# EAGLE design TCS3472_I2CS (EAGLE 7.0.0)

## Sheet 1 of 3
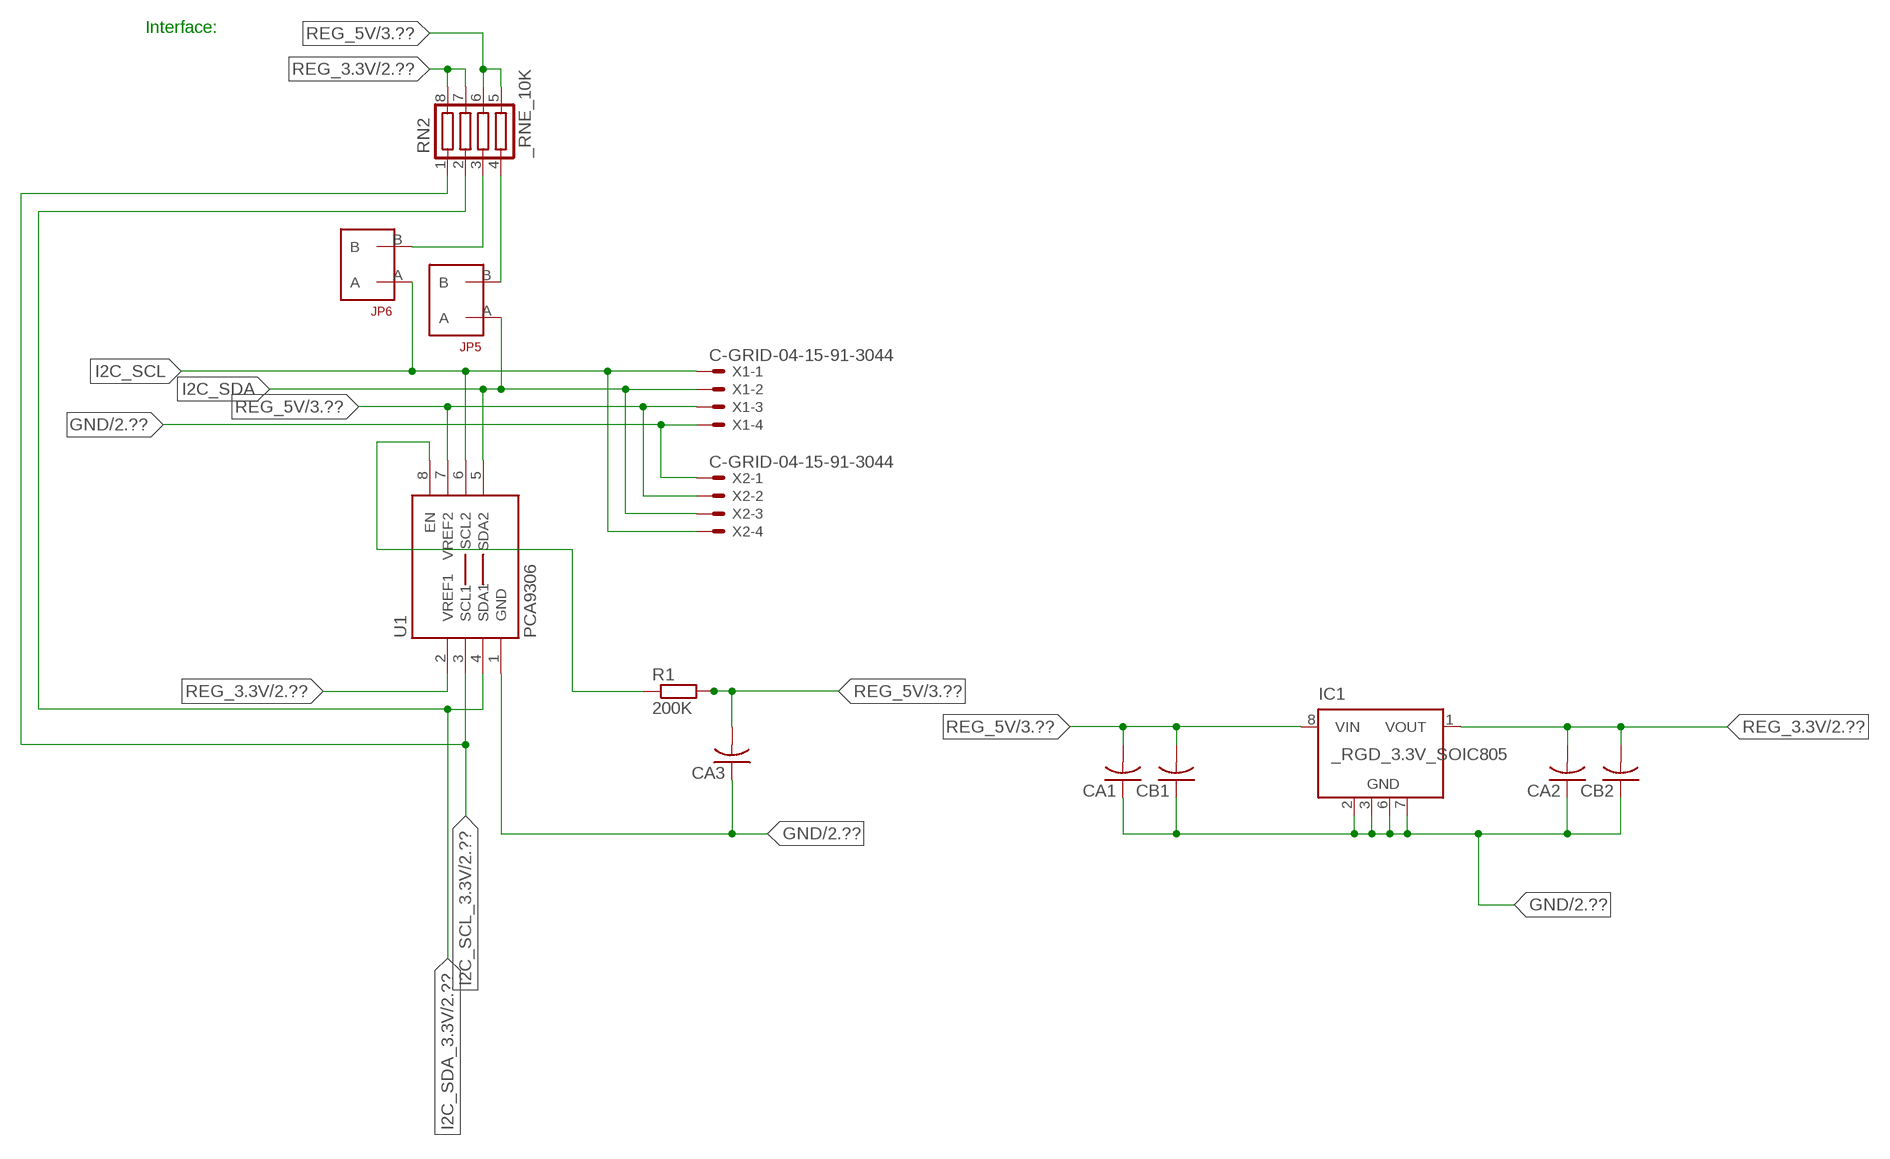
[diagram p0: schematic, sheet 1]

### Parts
CA1  CC1206KRX7R9BB104  [.1UF]
CA2  CC1206KRX7R9BB104  [.1UF]
CA3  CC1206KRX7R9BB104  [.1UF]
CB1  TMK316F106ZL-TC1206K  [TMK316F106ZL-T]
CB2  TMK316F106ZL-TC1206K  [TMK316F106ZL-T]
IC1  _RGD_3.3V_SOIC805  [_RGC_3.3V_SOIC8]
JP5  JUMPER_1X2_2MM  [JUMPER_1X2_2MM]
JP6  JUMPER_1X2_2MM  [JUMPER_1X2_2MM]
R1  200K  RESISTOR_SMT-0603  [R603]
RN2  _RNE_10K  [RNE]
U1  PCA9306  PCA9306_NCD  [PSOP-8]
X1  C-GRID-04-15-91-3044  [15-91-04]
X2  C-GRID-04-15-91-3044  [15-91-04]

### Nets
GND: CA1.1 CA2.1 CA3.1 CB1.1 CB2.1 IC1.2(GND) IC1.3(GND) IC1.6(GND) IC1.7(GND) U1.1(GND) X1.4 X2.1 ; also sheet 2,3
I2C_SCL: JP6.A U1.6(SCL2) X1.1 X2.4
I2C_SCL_3.3V: RN2.1 U1.3(SCL1) ; also sheet 2
I2C_SDA: JP5.A U1.5(SDA2) X1.2 X2.3
I2C_SDA_3.3V: RN2.2 U1.4(SDA1) ; also sheet 2
N$1: JP6.B RN2.3
N$2: JP5.B RN2.4
N$23: R1.1 U1.8(EN)
REG_3.3V: CA2.2 CB2.2 IC1.1(VOUT) RN2.7 RN2.8 U1.2(VREF1) ; also sheet 2
REG_5V: CA1.2 CA3.2 CB1.2 IC1.8(VIN) R1.2 RN2.5 RN2.6 U1.7(VREF2) X1.3 X2.2 ; also sheet 3
Unconnected: IC1.4(NC) IC1.5(NC)

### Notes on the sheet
- Interface:

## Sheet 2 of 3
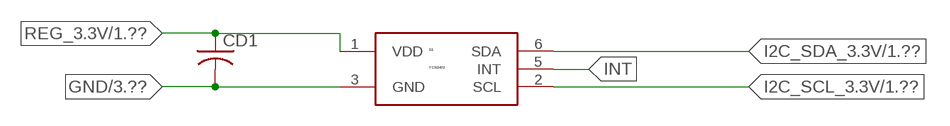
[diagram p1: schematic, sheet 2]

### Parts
CD1  CC1206KRX7R9BB103C1206K  [CC1206KRX7R9BB103]
S1  TCS3472  [FN-6]

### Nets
GND: CD1.2 S1.3(GND) ; also sheet 1,3
I2C_SCL_3.3V: S1.2(SCL) ; also sheet 1
I2C_SDA_3.3V: S1.6(SDA) ; also sheet 1
INT: S1.5(INT)
REG_3.3V: CD1.1 S1.1(VDD) ; also sheet 1

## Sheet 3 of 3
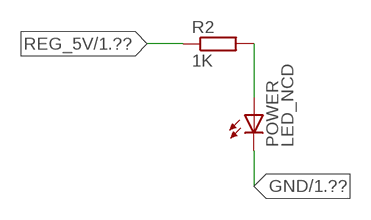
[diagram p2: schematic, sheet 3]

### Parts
POWER  LED_NCD  [CHIPLED_0603]
R2  1K  RESISTOR_SMT-0402  [R402]

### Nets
GND: POWER.C ; also sheet 1,2
N$4: POWER.A R2.2
REG_5V: R2.1 ; also sheet 1

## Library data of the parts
CA1-CA3 = NCD_ULTIMATE_LIBRARY:CC1206KRX7R9BB104: Capacitor CA .1uF 50V SMT C1206K CC1206KRX7R9BB104
CB1 CB2 = NCD_ULTIMATE_LIBRARY:TMK316F106ZL-T: Capacitor CB 10uF SMT 1206 TMK316F106ZL-T
CD1 = NCD_ULTIMATE_LIBRARY:CC1206KRX7R9BB103: Capacitor CD .01uF SMT CC1206KRX7R9BB103 1206
IC1 = NCD_ULTIMATE_LIBRARY:_RGD_3.3V_SOIC8: Regulator Linear 3.3V Chip Positive VOLTAGE REGULATOR Digikey 497-1199-2-ND/L78L33ACD13TR
JP5 JP6 = NCD_ULTIMATE_CONNECTORS:JUMPER_1X2_2MM
POWER = NCD_ULTIMATE_LIBRARY:LED_NCD: LED Digikey 754-1132-2-ND/APT2012SRCPRV
R1 R2 = NCD_ULTIMATE_LIBRARY:RESISTOR_SMT: NCD Resistor
RN2 = NCD_ULTIMATE_LIBRARY:_RNE_10K: Resistor Array RNE SMT 10K x 4 Single Resistor Source: http://www.ctscorp.com/components/Datasheets/CTSChipArrayDs.pdf Digikey 742C083103JPTR-ND/742C083103JP; OC_FARNELL: unknown; OC_NEWARK: unknown
S1 = NCD_ULTIMATE_bhaskar:TCS3472: Color Sensor Digikey TCS34725FNTR-ND/TCS34725FN
U1 = NCD_ULTIMATE_LIBRARY:PCA9306_NCD: NCD Bidirectional I2C level shifter. NOT compatible with all available part number pinout schemes- DOUBLE CHECK!!!; PROD_ID: IC-10023
X1 X2 = NCD_ULTIMATE_CONNECTORS:C-GRID-04: CONNECTOR 4-Pos I2C wire to board 2.54 mm (0.100") pitch header Digikey WM1342-ND/0015912045; OC_FARNELL: unknown; OC_NEWARK: unknown

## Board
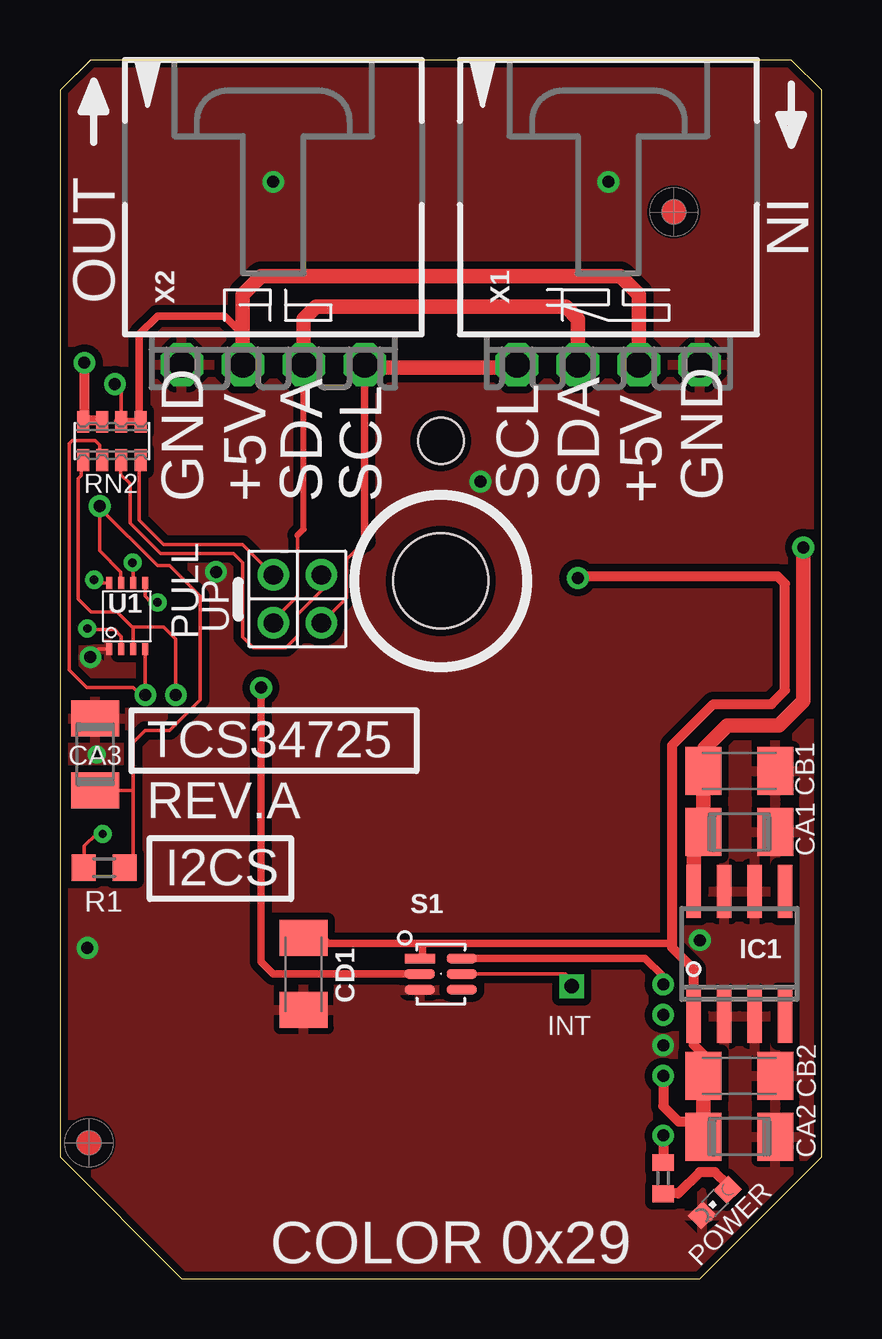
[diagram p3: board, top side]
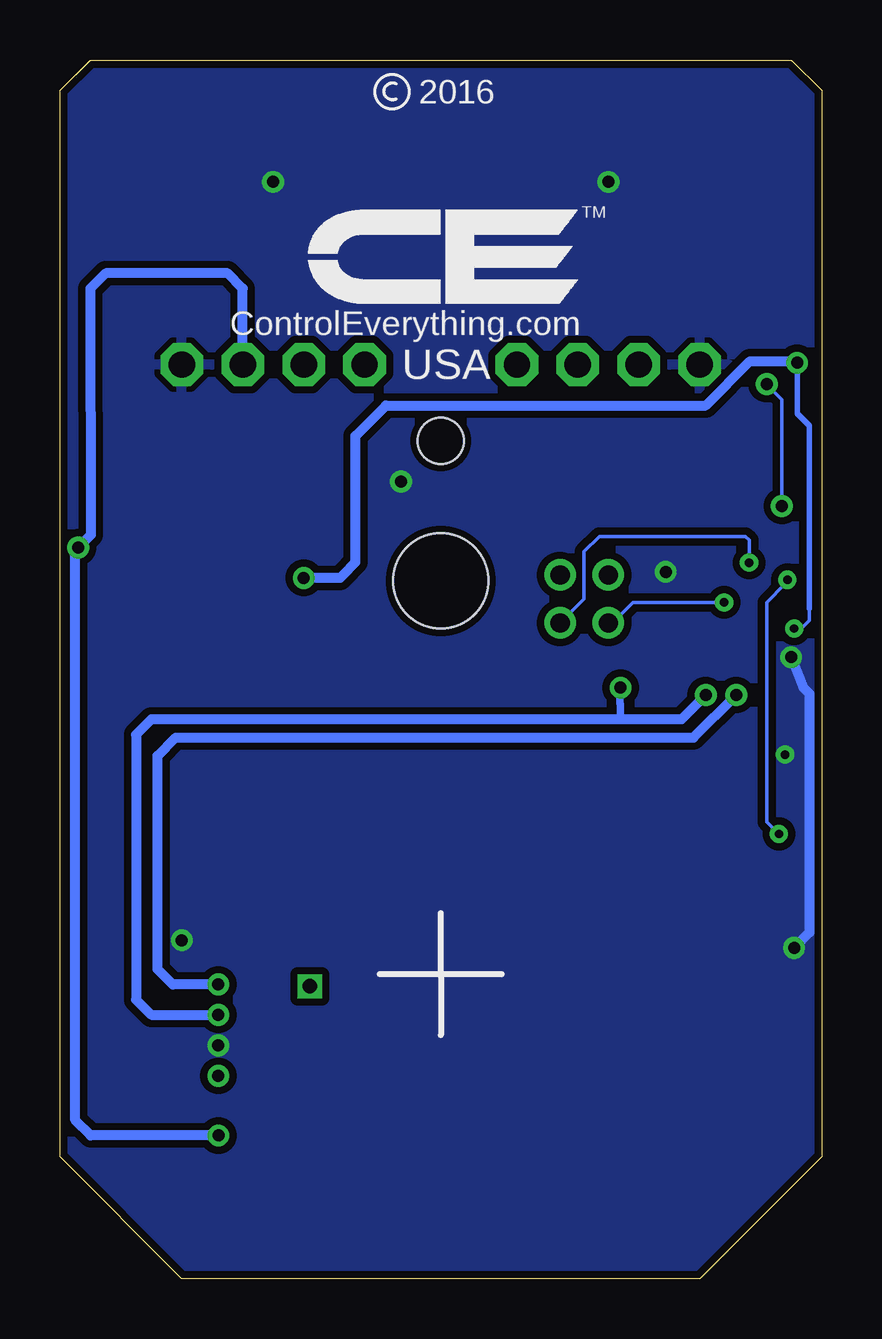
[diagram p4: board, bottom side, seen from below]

Size 31.75 x 50.8 mm. Coordinates in mm from the lower left corner, seen from the top.
Outline: 32 segments
Copper layers (1*16): Top 0.035mm / dielectric 1.5mm / Bottom 0.035mm
Design rules "default": minimum track width 5mil, minimum drill 24mil, track to track 5mil, track to pad 5mil, pad to pad 5mil, via to via 5mil, smd to smd 5mil, copper to edge 10mil, drill to drill 8mil, minimum pad ring 10mil, minimum via ring 8mil, stop-mask expansion 2mil, vias tented up to drill 0mil, thermal gap 10mil
Holes 3.96 mm at 15.88,29.08
Holes 1.91 mm at 15.88,34.93

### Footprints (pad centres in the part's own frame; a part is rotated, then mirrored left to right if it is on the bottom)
.1UF = smd 1.5 x 2: 1 -1.5,0; 2 1.5,0
TMK316F106ZL-T = smd 1.5 x 2: 1 -1.5,0; 2 1.5,0
CC1206KRX7R9BB103 = smd 1.5 x 2: 1 -1.5,0; 2 1.5,0
_RGC_3.3V_SOIC8 = smd 0.6 x 2.2: 1 -1.905,-2.6; 2 -0.635,-2.6; 3 0.635,-2.6; 4 1.905,-2.6; 5 1.905,2.6; 6 0.635,2.6; 7 -0.635,2.6; 8 -1.905,2.6
JUMPER_1X2_2MM = drill 0.8: A 0,2; B 0,0
CHIPLED_0603 = smd 0.8 x 0.876: A 0,-0.75; C 0,0.75
R603 = smd 1 x 1.1: 1 -0.85,0; 2 0.85,0
R402 = smd 0.7 x 0.9: 1 -0.65,0; 2 0.65,0
RNE = smd 0.5 x 0.9: 1 -1.2,-0.8; 2 -0.4,-0.8; 3 0.4,-0.8; 4 1.2,-0.8; 5 1.2,0.8; 6 0.4,0.8; 7 -0.4,0.8; 8 -1.2,0.8
FN-6 = smd 1.25 x 0.4: 1 -0.875,0.65; 2 -0.875,0; 3 -0.875,-0.65; 4 0.875,-0.65; 5 0.875,0; 6 0.875,0.65
PSOP-8 = smd 0.25 x 0.5: 1 -0.73,-1.37; 2 -0.23,-1.37; 3 0.27,-1.37; 4 0.77,-1.37; 5 0.77,1.38; 6 0.27,1.38; 7 -0.23,1.38; 8 -0.73,1.38
15-91-04 = drill 1.1 pad 1.778 octagon: 1 -3.81,-7.62; 2 -1.27,-7.62; 3 1.27,-7.62; 4 3.81,-7.62

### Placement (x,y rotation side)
CA1  28.32,18.62 180 top
CA2  28.32,5.92 180 top
CA3  1.46,21.86 270 top
CB1  28.32,21.16 180 top
CB2  28.32,8.46 180 top
CD1  10.16,12.7 270 top
IC1  28.32,13.54 0 top
JP5  8.89,29.34 180 top
JP6  10.9,29.34 180 top
POWER  27.3,3.18 135 top
R1  1.84,17.13 0 top
R2  25.15,4.19 270 top
RN2  2.16,34.93 0 top
S1  15.88,12.7 0 top
U1  2.79,27.61 0 top
U$5  [VISION_REF10]  1.21,5.66 90 top
U$28  [VISION_REF10]  25.59,44.46 90 top
X1  22.86,45.72 0 top
X2  8.89,45.72 0 top

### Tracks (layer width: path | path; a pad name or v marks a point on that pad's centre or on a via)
GND  (via drill 0.35, 0.5)
  Top 0.152: CA3.1 1.52,23.42 1.52,23.62 | v1.27,25.91 1.6,26.24 U1.1
  Bottom 0.406: v1.27,25.91 0.76,24.64 0.51,24.38 0.51,14.43 v1.15,13.79
  other vias: 8.89,45.72 22.86,45.72 25.15,9.73 17.53,33.22 26.67,14.11 6.5,29.46 1.52,21.84
  pour Bottom (isolate 0.305): -0.64,5.08 -0.64,49.53 1.27,51.44 30.48,51.44 32.38,49.53 32.38,5.08 26.67,-0.63 5.08,-0.63
  pour Top (isolate 0.305): 4.45,-1.27 -1.27,4.45 -1.27,50.17 0.64,52.07 31.11,52.07 33.02,50.17 33.02,4.45 27.3,-1.27
I2C_SCL  (via drill 0.35)
  Top 0.152: 12.7,30.73 11.94,29.97 11.94,28.38 JP6.A | v3.02,29.85 3.06,29.81 U1.6
  Top 0.305: 12.7,30.73 X2.4
  Top 0.406: X2.4 12.7,37.97 | 19.05,37.97 X1.1
  Top 0.61: 12.7,37.97 19.05,37.97
  Bottom 0.152: JP6.A 9.91,28.33 9.91,30.3 9.27,30.94 3.17,30.94 3.02,30.79 v3.02,29.85
I2C_SCL_3.3V  (via drill 0.5)
  Top 0.152: RN2.1 0.89,34.07 0.89,33.48 0.77,33.35 0.77,28.33 1.31,27.79 2.39,27.79 3.01,27.17 3.06,27.17 | 3.06,27.17 U1.3 | v4.83,24.33 v4.83,24.34 4.83,26.67 4.33,27.17 3.06,27.17
  Top 0.305: S1.2 8.89,12.7 8.38,13.21 v8.38,24.64
  Bottom 0.305: v8.38,24.64 8.41,24.61 8.41,23.98 8.38,23.95 8.38,23.32
  Bottom 0.406: v4.83,24.33 5.84,23.32 8.38,23.32 27.94,23.32 28.58,22.68 28.58,11.63 27.94,11 v25.15,11
I2C_SDA  (via drill 0.35)
  Top 0.152: JP5.A 8.89,27.44 9.91,28.45 9.91,30.99 | U1.5 3.56,28.45 3.81,28.19 v4.06,28.19
  Top 0.254: 9.91,30.99 10.16,31.25 X2.3
  Top 0.61: X2.3 10.16,40.01 10.67,40.51 21.09,40.51 21.59,40.01 X1.2
  Bottom 0.152: v4.06,28.19 7.87,28.19 8.73,27.34 JP5.A
I2C_SDA_3.3V  (via drill 0.5)
  Top 0.152: RN2.2 1.65,34.14 1.65,34.75 1.46,34.94 0.51,34.94 0.38,34.81 0.38,26.37 0.38,26.36 0.38,25.38 1.12,24.64 3.05,24.64 3.35,24.33 v3.56,24.33 v3.56,24.34 U1.4
  Top 0.305: S1.6 24.38,13.36 25.15,12.6 v25.15,12.27
  Bottom 0.406: v25.15,12.27 27.05,12.27 27.69,12.9 27.69,21.79 26.93,22.56 5.34,22.56 v3.56,24.33
INT  (via drill 0.6)
  Top 0.152: S1.5 21.08,12.7 21.34,12.45 v21.34,12.19
N$1
  Top 0.152: JP6.B 10.92,29.31 10.92,28.7 9.91,27.69 9.91,26.8 9.42,26.31 8.06,26.31 7.62,26.75 7.62,29.84 7.24,30.23 4.19,30.23 2.92,31.5 2.92,33.15 2.54,33.53 2.54,34.1 RN2.3
  Top 0.305: 2.54,34.02 RN2.3
N$2
  Top 0.152: JP5.B 7.62,30.61 4.32,30.61 3.3,31.62 3.3,34.07 RN2.4
  Top 0.305: 3.37,33.88 RN2.4
N$4
  Top 0.406: POWER.A 27.84,3.92 27.3,4.45 26.67,4.45 25.78,3.56 25.16,3.56 R2.2
N$23  (via drill 0.35)
  Top 0.152: R1.1 1.02,17.16 1.02,18.03 1.52,18.54 v1.78,18.54 | v1.42,29.13 1.74,28.99 U1.8
  Bottom 0.152: v1.78,18.54 2.29,19.05 2.29,28.19 1.52,28.96 v1.42,29.13
REG_3.3V  (via drill 0.35, 0.5)
  Top 0.152: v1.14,27.1 1.19,27.05 2.29,27.05 2.56,26.78 U1.2
  Top 0.305: 15.11,13.97 11.18,13.97 10.95,14.2 CD1.1 | 15.11,13.97 25.53,13.97 | S1.1 15.11,13.46 15.11,13.97
  Top 0.406: CB2.2 26.82,9.35 26.42,9.75 26.42,10.36 | v25.15,8.46 25.15,7.19 25.78,6.55 26.82,6.55 | IC1.1 26.42,12.9 25.53,13.79 25.53,13.97 25.53,22.24 27.24,23.95 29.66,23.95 30.23,24.52 30.23,28.97 29.91,29.29 21.67,29.29 v21.59,29.21 | 26.52,5.62 CA2.2 | v1.02,38.18 1.02,35.78 | 1.02,35.78 RN2.8 | 1.02,35.78 1.71,35.78 RN2.7
  Top 0.61: CB2.2 26.82,6.55 CA2.2 | 26.42,10.36 IC1.1
  Bottom 0.152: 0.51,27.94 0.51,27.43 0.84,27.1 v1.14,27.1
  Bottom 0.229: 0.51,27.94 0.51,35.56 1.02,36.07 v1.02,38.18
  Bottom 0.406: v1.02,38.18 1.08,38.24 2.99,38.24 4.83,36.4 18.16,36.4 19.43,35.13 19.43,29.87 19.94,29.34 20.07,29.21 v21.59,29.21
REG_5V  (via drill 0.5)
  Top 0.152: RN2.6 2.56,37.01 v2.29,37.29 | R1.2 3.05,17.49 3.05,20.36 | 3.05,20.36 3.05,22.35 3.56,22.86 4.57,22.86 5.84,24.13 5.84,28.45 4.57,29.72 4.06,29.72 1.65,32.13 v1.65,32.21 1.65,30.35 2.54,29.46 2.54,29.01 U1.7 | CA3.2 3.05,20.36
  Top 0.305: 7.62,39.37 7.5,39.37 | 2.42,35.74 RN2.6 RN2.5 3.31,35.8 3.31,39.37 4.07,40.13 6.86,40.13 7.62,39.37 | X2.2 7.62,39.37
  Top 0.406: v25.15,5.97 R2.1
  Top 0.61: X1.3 24.13,38.23 24.13,41.02 23.37,41.78 8.38,41.78 7.62,41.02 X2.2 | IC1.8 26.42,18.21 CA1.2 CB1.2 26.86,21.2 26.86,22.11 27.82,23.06 29.98,23.06 30.99,24.08 v30.99,30.48
  Bottom 0.152: v1.65,32.21 1.65,36.65 v2.29,37.29
  Bottom 0.406: X1.3 24.13,41.28 24.77,41.91 29.84,41.91 30.48,41.27 30.47,31 v30.99,30.48 31.11,30.36 31.11,6.6 30.48,5.97 v25.15,5.97

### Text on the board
tPlace: COLOR 0x29
tNames: IN | OUT | GND | +5V | SDA | SCL | SCL | SDA | +5V | GND | PULL | UP | TCS34725 | REV.A | I2CS | INT
bNames: 2016 | TM | ControlEverything.com | USA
